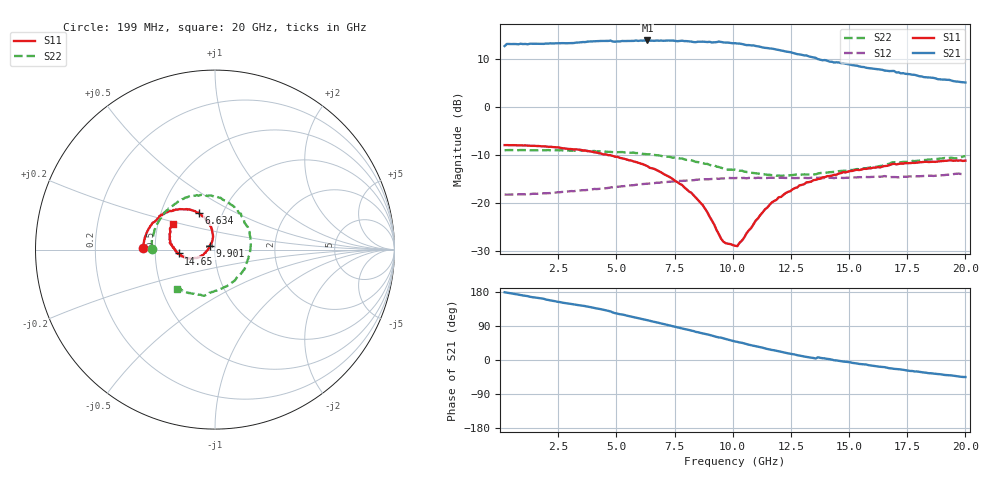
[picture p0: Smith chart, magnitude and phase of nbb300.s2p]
!  File: NBB300
!  Wafer #: rf nitro
!  Device #:
!  Frequency sweeps: 201
!  Date:  7 Aug 2001
!  Time: 15:57:50
!  Gate Voltage(V): +0.00  Gate Current(uA):  +0.00
!  Drain Voltage(V): +0.00  Drain Current(mA):  +0.00
# GHZ S DB R 50
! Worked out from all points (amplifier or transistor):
!   201 points, 199 MHz to 20 GHz, reference 50 ohm
!   highest |S21| = 13.9 dB at 6.337 GHz (marker M1)
!   |S21| within 3 dB of that: start of sweep to 12.97 GHz
!   unconditionally stable (mu >= 1): start of sweep to 4.462 GHz; 10.46 GHz to end of sweep
!   at 3.466 GHz: K = 1.02, MAG = 14.6 dB, |S12| = -17.4 dB
!   at 10.1 GHz: K = 0.99, MSG = 14.1 dB, |S12| = -14.9 dB
!   at 20 GHz: K = 1.36, MAG = 6.0 dB, |S12| = -14.0 dB
!   S11 on the Smith chart (normalised r, x): 199 MHz: 0.43, +0.01; 6.634 GHz: 0.77, +0.33; 9.901 GHz: 0.94, +0.04; 14.65 GHz: 0.66, -0.03; 20 GHz: 0.60, +0.19
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0.199  -7.95 178.9  12.75 178.8  -18.29 0.1  -9.03 179.3
0.29801  -7.95 178.0  13.20 177.7  -18.31 0.4  -9.01 178.3
0.89204  -8.00 172.4  13.24 171.1  -18.24 1.4  -8.99 172.7
3.56517  -9.09 146.9  13.59 143.1  -17.38 3.5  -9.13 146.6
4.75323  -10.08 134.4  13.90 128.2  -16.82 2.7  -9.41 132.6
4.95124  -10.38 132.4  13.67 123.5  -16.70 2.2  -9.45 130.1
6.33731  -12.37 117.2  13.92 104.9  -16.01 -0.8  -9.89 110.0
6.63433  -12.94 114.0  13.84 100.7  -15.91 -1.7  -10.03 105.4
6.83234  -13.42 112.8  13.87 97.8  -15.83 -2.5  -10.11 102.0
7.82239  -16.29 103.3  13.87 83.4  -15.45 -5.5  -10.75 83.7
9.40647  -26.60 111.0  13.69 59.6  -15.02 -11.5  -12.55 49.2
9.90149  -28.66 144.2  13.39 51.7  -14.84 -13.8  -13.08 39.9
10.0995  -28.99 160.0  13.35 49.0  -14.87 -14.4  -13.07 34.3
10.89154  -24.51 -162.1  12.89 37.5  -14.79 -17.6  -13.78 12.9
11.68358  -19.95 -154.2  12.23 26.5  -14.78 -20.3  -14.24 -7.8
12.77264  -16.83 -159.9  11.06 12.8  -14.84 -23.3  -14.08 -34.1
13.46567  -15.29 -165.9  10.37 5.4  -14.77 -25.2  -14.09 -50.4
13.56468  -15.22 -165.2  10.29 3.8  -14.78 -25.5  -14.07 -52.8
13.66368  -15.06 -166.1  10.02 7.3  -14.80 -25.8  -13.91 -54.6
14.65373  -13.83 -174.0  9.18 -3.0  -14.78 -27.6  -13.36 -73.2
16.73284  -12.15 173.4  7.51 -21.8  -14.67 -33.8  -11.83 -100.8
20  -11.20 148.4  5.13 -45.0  -14.03 -40.0  -10.26 -134.3
